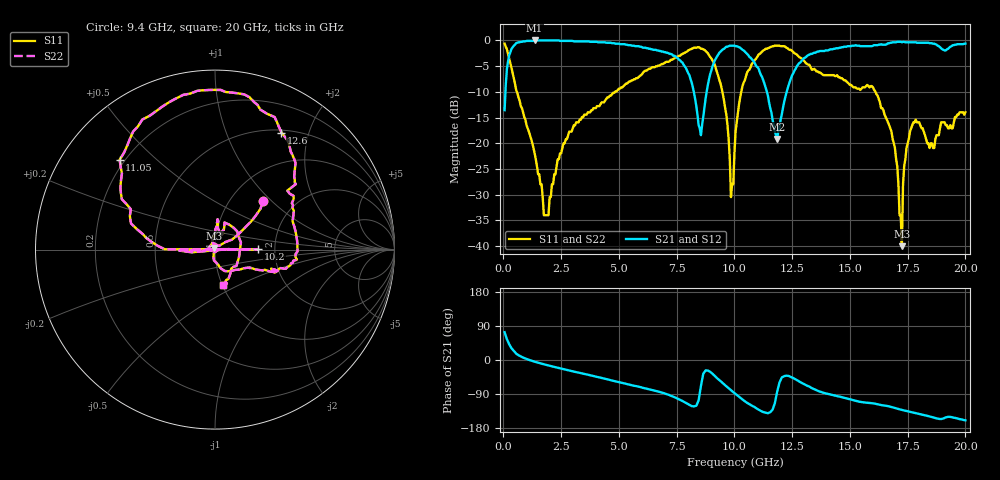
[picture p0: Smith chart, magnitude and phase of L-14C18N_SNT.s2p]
#	mhz	s	ma	r	50
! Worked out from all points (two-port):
!   400 points, 50 MHz to 20 GHz, reference 50 ohm
!   highest |S21| = 0.00 dB at 1.35 GHz (marker M1); lowest = -19.2 dB at 11.85 GHz (marker M2)
!   |S21| within 3 dB of the highest: 243.7 MHz to 7.41 GHz (7.167 GHz wide, 187 % of centre); 13.14 GHz to end of sweep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
!   lowest |S11| = -40.0 dB at 17.25 GHz (marker M3), VSWR 1.02, Z = 49.7 + j0.935 ohm
!   |S11| at or under -10 dB: 584.1 MHz to 4.831 GHz (4.247 GHz wide, 157 % of centre); 9.479 GHz to 10.3 GHz (816.6 MHz wide, 8.26 % of centre); 16.11 GHz to end of sweep
!   |S22| runs from -40.0 to -0.6 dB; largest |S21 - S12| = 0
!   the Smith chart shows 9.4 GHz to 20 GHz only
!   S11 on the Smith chart (normalised r, x): 9.4 GHz: 1.41, +0.89; 10.2 GHz: 1.63, +0.01; 11.05 GHz: 0.18, +0.39; 12.6 GHz: 0.53, +1.59; 20 GHz: 1.01, -0.41
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50  0.93 167.0  0.21 73.2  0.21 73.2  0.93 167.0
1350  0.08 72.2  1 -4.5  1 -4.5  0.08 72.2
1950  0.02 -45.7  1 -14.3  1 -14.3  0.02 -45.7
3400  0.18 -120.5  0.98 -35.4  0.98 -35.4  0.18 -120.5
6700  0.57 -174.8  0.8 -83.3  0.8 -83.3  0.57 -174.8
6850  0.59 -178.6  0.78 -86.0  0.78 -86.0  0.59 -178.6
6900  0.59 0.6  0.78 -86.8  0.78 -86.8  0.59 0.6
6950  0.6 179.9  0.77 -87.6  0.77 -87.6  0.6 179.9
7050  0.62 176.5  0.76 -89.9  0.76 -89.9  0.62 176.5
8550  0.83 103.3  0.12 -68.6  0.12 -68.6  0.83 103.3
9400  0.38 45.2  0.78 -55.8  0.78 -55.8  0.38 45.2
9850  0.03 42.6  0.89 -79.7  0.89 -79.7  0.03 42.6
10050  0.13 -173.4  0.88 -89.8  0.88 -89.8  0.13 -173.4
10200  0.24 0.5  0.86 -96.9  0.86 -96.9  0.24 0.5
11050  0.73 136.7  0.53 -131.2  0.53 -131.2  0.73 136.7
11850  0.89 92.3  0.11 -83.7  0.11 -83.7  0.89 92.3
12600  0.75 60.4  0.51 -49.5  0.51 -49.5  0.75 60.4
13350  0.52 39.2  0.74 -74.2  0.74 -74.2  0.52 39.2
16700  0.15 -52.3  0.94 -122.5  0.94 -122.5  0.15 -52.3
17250  0.01 109.7  0.96 -131.6  0.96 -131.6  0.01 109.7
17750  0.16 83.9  0.96 -138.7  0.96 -138.7  0.16 83.9
20000  0.2 -77.4  0.93 -159.1  0.93 -159.1  0.2 -77.4
